PROGRAM MAIN
VAR
	b_pfail AT %I*: BOOL;								//用于接收CU8130-0120的P FAIL口输出的关闭Uin的输入电压
	b_upsen AT %Q*: BOOL:= TRUE;						//用于给CU8130-0120的UPS EN	口输入高电平，当P Fail口有输出时给UPS EN口一个下降沿用于关闭U1,2out的输出
	b_upsready AT %I*:BOOL;
	FB_WritePersistentData: FB_WritePersistentData;		//该功能块用于写入持续的数据起到掉电数据保存的功能
	b_start: BOOL;
	b_busy: BOOL;
	FB_TON: TON;
	b_PSHDN AT %Q*: BOOL;
END_VAR
VAR PERSISTENT
	Array_persistent: ARRAY[0..1048575] OF byte;
END_VAR

FB_WritePersistentData(
	NETID:= , 
	PORT:= 852, 
	START:= b_start, 
	TMOUT:= , 
	MODE:= , 
	BUSY=> b_busy, 
	ERR=> , 
	ERRID=> );
FB_TON(IN:= , PT:= T#15S, Q=> , ET=> );
IF b_pfail=TRUE THEN
	b_start:=TRUE;
	IF NOT(b_busy=TRUE) THEN
		FB_TON.IN:=TRUE;
		IF FB_TON.Q=TRUE THEN
			b_upsen:=FALSE;
		END_IF
	END_IF
ELSE b_upsen:=TRUE;
END_IF

END_PROGRAM
